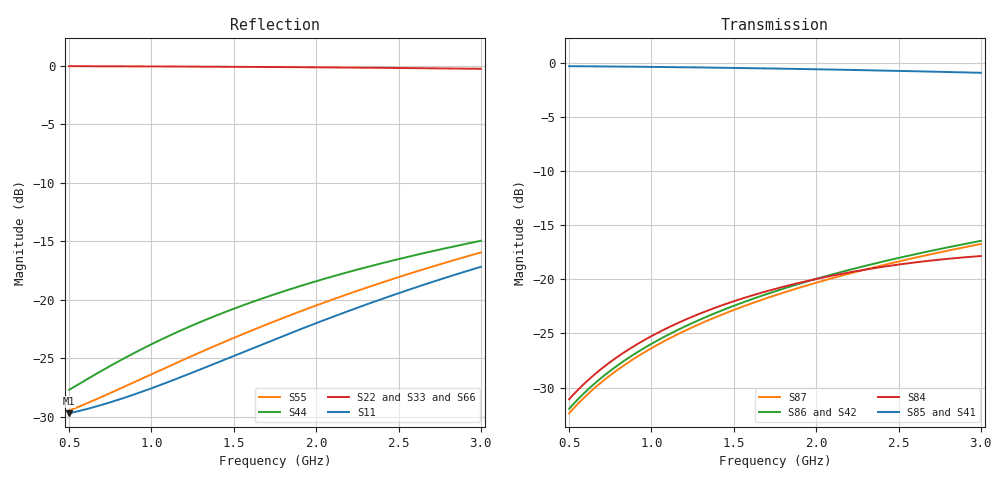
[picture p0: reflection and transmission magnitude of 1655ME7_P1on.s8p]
! Created Fri Dec 10 20:15:46 2010
# hz S db R 50
! 8 Port Network Data from SP1.SP block
! freq  dbS11  angS11  dbS12  angS12  dbS13  angS13  dbS14  angS14
!  dbS15  angS15  dbS16  angS16  dbS17  angS17  dbS18  angS18
!  dbS21  angS21  dbS22  angS22  dbS23  angS23  dbS24  angS24
!  dbS25  angS25  dbS26  angS26  dbS27  angS27  dbS28  angS28
!  dbS31  angS31  dbS32  angS32  dbS33  angS33  dbS34  angS34
!  dbS35  angS35  dbS36  angS36  dbS37  angS37  dbS38  angS38
!  dbS41  angS41  dbS42  angS42  dbS43  angS43  dbS44  angS44
!  dbS45  angS45  dbS46  angS46  dbS47  angS47  dbS48  angS48
!  dbS51  angS51  dbS52  angS52  dbS53  angS53  dbS54  angS54
!  dbS55  angS55  dbS56  angS56  dbS57  angS57  dbS58  angS58
!  dbS61  angS61  dbS62  angS62  dbS63  angS63  dbS64  angS64
!  dbS65  angS65  dbS66  angS66  dbS67  angS67  dbS68  angS68
!  dbS71  angS71  dbS72  angS72  dbS73  angS73  dbS74  angS74
!  dbS75  angS75  dbS76  angS76  dbS77  angS77  dbS78  angS78
!  dbS81  angS81  dbS82  angS82  dbS83  angS83  dbS84  angS84
!  dbS85  angS85  dbS86  angS86  dbS87  angS87  dbS88  angS88
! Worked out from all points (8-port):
!   251 points, 500 MHz to 3 GHz, reference 50 ohm
!   strongest paths, dB at 500 MHz, 1.12 GHz, 1.75 GHz, 2.38 GHz, 3 GHz:
!     S85: -0.3, -0.4, -0.5, -0.7, -0.9
!     S41: -0.3, -0.4, -0.5, -0.7, -0.9
!     S84: -31.1, -24.3, -20.9, -18.9, -17.9
!     S86: -32.0, -25.0, -21.1, -18.5, -16.4
!     S42: -32.1, -25.1, -21.2, -18.5, -16.5
!     S87: -32.4, -25.4, -21.5, -18.8, -16.7
!   lowest |S11| = -29.7 dB at 500 MHz (marker M1), VSWR 1.07, Z = 52.4 - j2.36 ohm
!   |S11| at or under -10 dB: start of sweep to end of sweep
